{attribute 'no_assign'}
FUNCTION_BLOCK FB_DO_IED_MUnn_InnATCTR1_AmpSv EXTENDS FB_AcsiCommonDataClass
VAR_INPUT
	instMag: FB_AcsiDATypeAnalogueValue := (Fc:=ACSI_FC_MX, f:=(bPresence:=FALSE), bLinkResult:=THIS^.AddDataToContainer(ipData:=instMag));
	q: FB_AcsiDATypeQuality := (Fc:=ACSI_FC_MX, TrgOp:=ACSI_TrgOp_qchg, bLinkResult:=THIS^.AddDataToContainer(ipData:=q));
	units: FB_AcsiDATypeUnit := (Fc:=ACSI_FC_CF, TrgOp:=ACSI_TrgOp_dchg, SIUnit:=(eValue:=E_AcsiSIUnit.Ampere), multiplier:=(eValue:=E_AcsiMultiplier.Kilo, bPresence:=TRUE), bLinkResult:=THIS^.AddDataToContainer(ipData:=units));
	sVC: FB_AcsiDATypeScaledValueConfig := (Fc:=ACSI_FC_CF, TrgOp:=ACSI_TrgOp_dchg, scaleFactor:=(fValue:=0.001), bLinkResult:=THIS^.AddDataToContainer(ipData:=sVC));
END_VAR
VAR
END_VAR

END_FUNCTION_BLOCK
